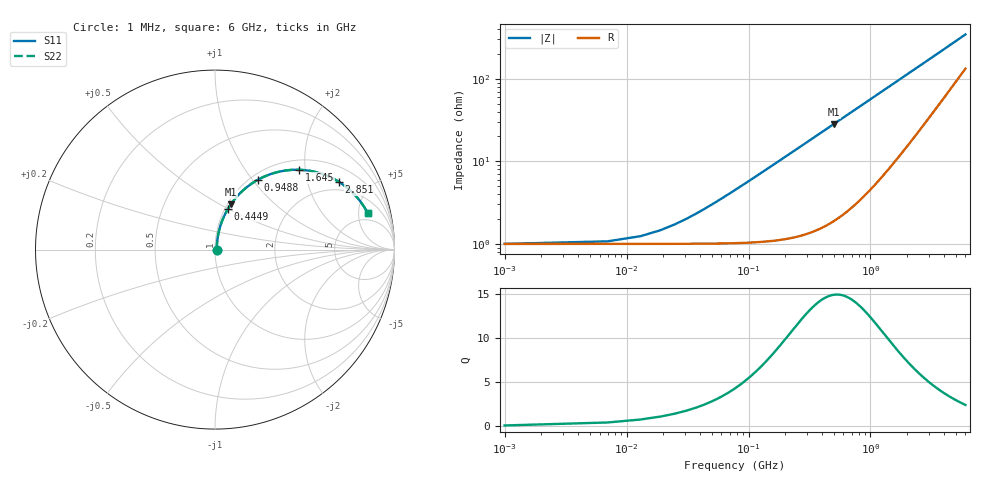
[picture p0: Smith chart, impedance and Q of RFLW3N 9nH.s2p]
!Vishay Electro-Films
!RFLW3N9000C - 9 nH Spiral Inductor on Quartz
!Measured in series configuration
!May 2011
# GHz S MA R 50
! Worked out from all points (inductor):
!   1001 points, 1 MHz to 6 GHz, reference 50 ohm
!   read as one part in series: L = 8.98 nH near 54.99 MHz
!   highest Q = 15 at 498.9 MHz (marker M1), where L = 8.98 nH
!   S11 on the Smith chart (normalised r, x): 1 MHz: 1.02, +0.00; 444.9 MHz: 1.03, +0.50; 948.8 MHz: 1.08, +1.07; 1.645 GHz: 1.21, +1.85; 2.851 GHz: 1.60, +3.18; 6 GHz: 3.65, +6.35
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0.001  0.009906 3.2  0.9901 -0.0  0.9901 -0.0  0.009906 3.2
0.018997  0.01451 46.4  0.99 -0.6  0.99 -0.6  0.01451 46.4
0.054991  0.03229 70.2  0.9895 -1.8  0.9895 -1.8  0.03229 70.2
0.072988  0.04196 73.8  0.9891 -2.3  0.9891 -2.3  0.04196 73.8
0.102983  0.05832 76.6  0.9881 -3.3  0.9881 -3.3  0.05832 76.6
0.144976  0.08136 77.9  0.9862 -4.6  0.9862 -4.6  0.08136 77.9
0.198967  0.1109 77.9  0.9827 -6.3  0.9827 -6.3  0.1109 77.9
0.270955  0.1498 76.7  0.9765 -8.6  0.9765 -8.6  0.1498 76.7
0.348942  0.191 74.9  0.9678 -11.0  0.9678 -11.0  0.191 74.9
0.444926  0.2401 72.3  0.9546 -13.9  0.9546 -13.9  0.2401 72.3
0.498917  0.2668 70.7  0.9461 -15.4  0.9461 -15.4  0.2668 70.7
0.702883  0.3607 64.9  0.908 -21.1  0.908 -21.1  0.3607 64.9
0.948842  0.4579 58.4  0.8539 -27.2  0.8539 -27.2  0.4579 58.4
1.00283  0.4769 57.0  0.8414 -28.4  0.8414 -28.4  0.4769 57.0
1.29678  0.5662 50.2  0.7722 -34.3  0.7722 -34.3  0.5662 50.2
1.64473  0.6454 43.6  0.6937 -39.9  0.6937 -39.9  0.6454 43.6
2.00467  0.7046 38.0  0.6209 -44.3  0.6209 -44.3  0.7046 38.0
2.85053  0.7875 28.6  0.4871 -50.7  0.4871 -50.7  0.7875 28.6
3.0005  0.797 27.3  0.4682 -51.4  0.4682 -51.4  0.797 27.3
4.00233  0.8395 20.9  0.3686 -54.2  0.3686 -54.2  0.8395 20.9
5.00417  0.8616 16.6  0.3015 -54.7  0.3015 -54.7  0.8616 16.6
6  0.8742 13.6  0.2542 -53.8  0.2542 -53.8  0.8742 13.6
